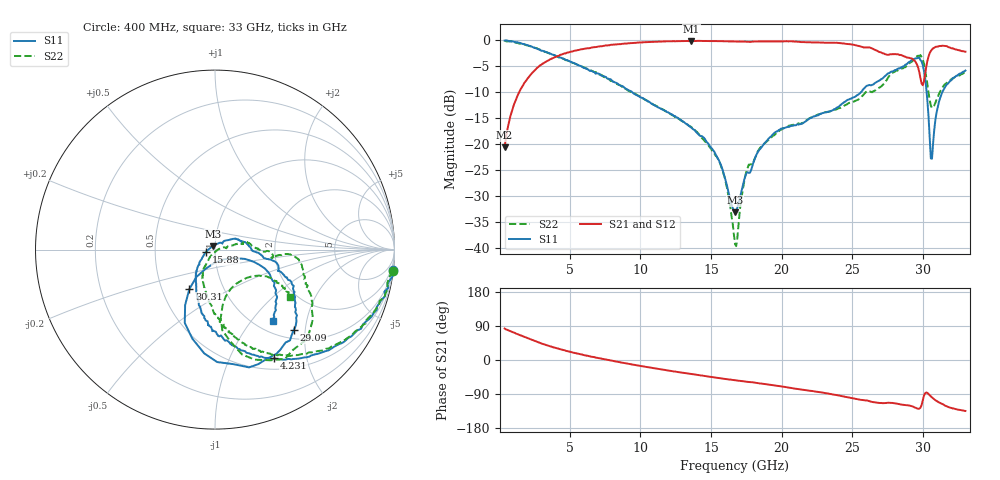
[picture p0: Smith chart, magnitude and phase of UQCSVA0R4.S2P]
!  Part Number  UQCSVA0R4  Mounting Orientation: Horizontal
!  Description: Ultra Low ESR Microwave capacitors
!  Application: Coupling, Bypass, Tuning, DC Block
!  Filters, Matching
# GHZ S DB R 50
! Freq  |S11|  S11 Ph  |S21|  S21 Ph  |S12|  S12 Ph  |S22|  S22 Ph
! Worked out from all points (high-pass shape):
!   401 points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, 400 MHz to 33 GHz, reference 50 ohm
!   highest |S21| = -0.08 dB at 13.6 GHz (marker M1); lowest = -20.6 dB at 400 MHz (marker M2)
!   |S21| within 3 dB of the highest: 4.084 GHz to 28.68 GHz (24.6 GHz wide, 150 % of centre); 30.39 GHz to end of sweep
!   lowest |S11| = -33.1 dB at 16.7 GHz (marker M3), VSWR 1.05, Z = 48.9 + j1.9 ohm
!   |S11| at or under -10 dB: 9.443 GHz to 25.6 GHz (16.15 GHz wide, 92.2 % of centre); 30.26 GHz to 31.36 GHz (1.103 GHz wide, 3.58 % of centre)
!   |S22| runs from -39.6 to 0.0 dB; largest |S21 - S12| = 0.014
!   S11 on the Smith chart (normalised r, x): 400 MHz: 0, -18; 4.231 GHz: 0.64, -1.49; 15.88 GHz: 0.90, -0.03; 29.09 GHz: 1.18, -1.74; 30.31 GHz: 0.69, -0.32; 33 GHz: 1.19, -1.29
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0.4  -0.02 -6.5  -20.61 83.0  -20.57 82.9  -0.01 -6.8
1.704  -0.69 -26.8  -8.65 62.5  -8.62 61.5  -0.69 -27.5
4.231  -3.22 -61.3  -2.97 29.5  -2.98 29.8  -3.28 -58.5
5.861  -5.05 -77.4  -1.71 14.5  -1.68 14.6  -5.01 -71.8
11.321  -12.96 -118.0  -0.22 -23.8  -0.20 -23.8  -12.91 -104.5
13.603  -16.77 -133.1  -0.08 -37.1  -0.11 -37.0  -16.67 -117.6
15.885  -25.51 -164.7  -0.15 -49.4  -0.15 -49.4  -25.67 -124.5
16.7  -33.06 119.2  -0.20 -53.4  -0.19 -53.4  -39.18 -70.2
16.863  -32.23 95.9  -0.20 -54.1  -0.21 -54.1  -38.16 -14.2
17.515  -25.54 45.1  -0.25 -57.5  -0.24 -57.4  -25.13 13.1
18.412  -21.08 36.5  -0.22 -61.6  -0.21 -61.6  -20.94 14.2
22.161  -14.85 10.0  -0.37 -81.8  -0.34 -81.8  -14.71 12.8
26.399  -8.55 -18.4  -1.53 -110.7  -1.54 -110.8  -9.97 -8.1
27.621  -6.28 -26.5  -2.72 -112.9  -2.74 -112.5  -6.80 -5.8
29.088  -4.06 -45.6  -3.41 -120.7  -3.37 -120.7  -4.28 -28.0
29.822  -3.79 -80.9  -7.30 -125.8  -7.14 -125.2  -2.82 -57.4
30.066  -5.81 -104.2  -7.90 -94.3  -7.77 -94.6  -4.39 -75.6
30.311  -11.64 -123.0  -3.95 -86.7  -3.94 -87.1  -8.37 -85.2
30.474  -18.58 -115.8  -2.43 -92.5  -2.44 -92.4  -11.40 -77.4
30.637  -22.77 -49.2  -1.73 -98.7  -1.75 -98.6  -12.99 -58.3
31.37  -9.93 -22.7  -1.01 -116.5  -1.02 -116.2  -9.08 -26.9
33  -5.80 -51.1  -2.16 -134.5  -2.18 -134.4  -6.16 -32.2
